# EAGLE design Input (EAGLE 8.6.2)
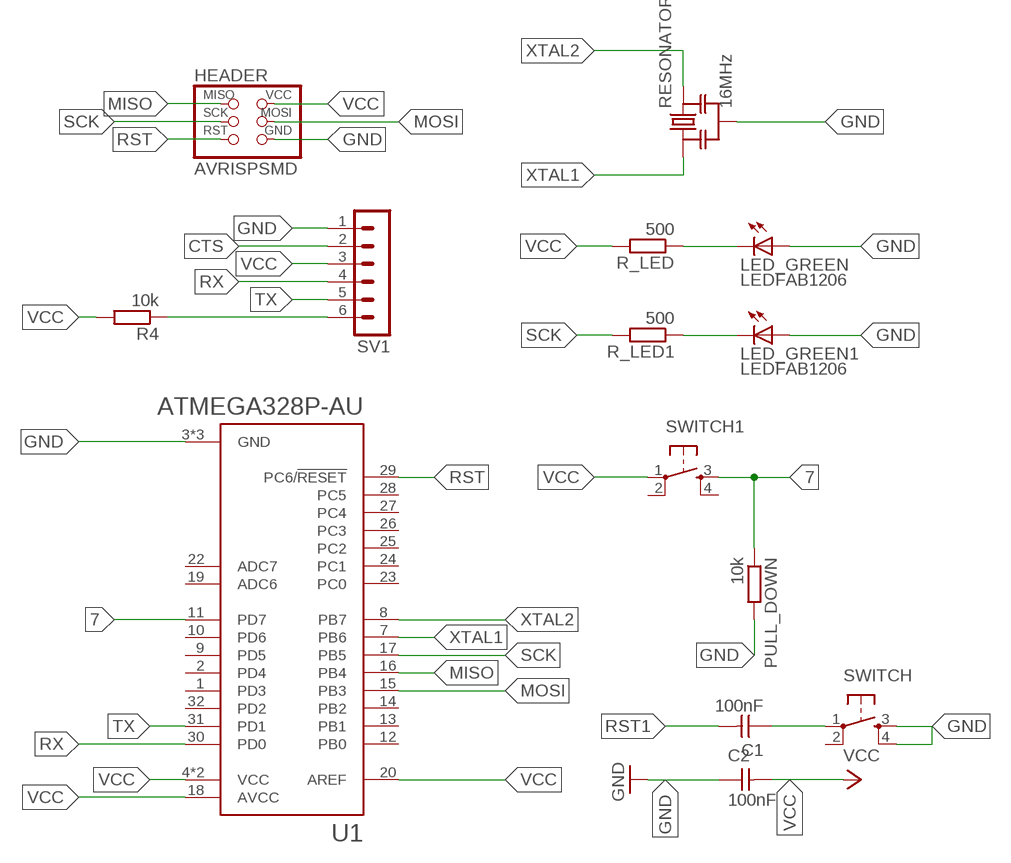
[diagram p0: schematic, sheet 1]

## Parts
C1  100nF  CAP-UNPOLARIZEDFAB  [C1206FAB]
C2  100nF  CAP-UNPOLARIZEDFAB  [C1206FAB]
HEADER  AVRISPSMD  [2X03SMD]
LED_GREEN  LEDFAB1206  [LED1206FAB]
LED_GREEN1  LEDFAB1206  [LED1206FAB]
PULL_DOWN  10k  R-EU_R1206  [R1206]
R4  10k  R-EU_R1206  [R1206]
R_LED  500  R-EU_R1206  [R1206]
R_LED1  500  R-EU_R1206  [R1206]
RESONATOR  16MHz  RESONATOR-MURATACSTCR_G  [RESONATOR_MURATA3]
SV1  MA06-1  [MA06-1]
SWITCH  6MM_SWITCH6MM_SWITCH  [6MM_SWITCH]
SWITCH1  6MM_SWITCH6MM_SWITCH  [6MM_SWITCH]
U1  ATMEGA328P-AU  [QFP80P900X900X120-32N]

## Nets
7: PULL_DOWN.1 SWITCH1.3(S) U1.11(PD7)
CTS: SV1.2
GND: C2.1 HEADER.6(GND) LED_GREEN1.1(A) LED_GREEN.1(A) PULL_DOWN.2 RESONATOR.2 SV1.1 SWITCH.3(S) SWITCH.4(S1) U1.3(GND) U1.5(GND) U1.21(GND)
MISO: HEADER.1(MISO) U1.16(PB4)
MOSI: HEADER.4(MOSI) U1.15(PB3)
N$1: LED_GREEN1.2(C) R_LED1.1
N$21: LED_GREEN.2(C) R_LED.1
RST: C1.1 HEADER.5(RST) SWITCH.1(P) U1.29(PC6/!RESET)
RST1: C1.2 R4.1 SV1.6
RX: SV1.4 U1.30(PD0)
SCK: HEADER.3(SCK) R_LED1.2 U1.17(PB5)
TX: SV1.5 U1.31(PD1)
VCC: C2.2 HEADER.2(VCC) R4.2 R_LED.2 SV1.3 SWITCH1.1(P) U1.4(VCC) U1.6(VCC) U1.18(AVCC) U1.20(AREF)
XTAL1: RESONATOR.1 U1.7(PB6)
XTAL2: RESONATOR.3 U1.8(PB7)
Unconnected: SWITCH1.2(P1) SWITCH1.4(S1) SWITCH.2(P1) U1.1(PD3) U1.2(PD4) U1.9(PD5) U1.10(PD6) U1.12(PB0) U1.13(PB1) U1.14(PB2) U1.19(ADC6) U1.22(ADC7) U1.23(PC0) U1.24(PC1) U1.25(PC2) U1.26(PC3) U1.27(PC4) U1.28(PC5) U1.32(PD2)

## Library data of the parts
C1 C2 = fab:CAP-UNPOLARIZED
HEADER = fab:AVRISP
LED_GREEN LED_GREEN1 = fab:LED: LED
PULL_DOWN R4 R_LED R_LED1 = resistor:R-EU_: RESISTOR, European symbol
RESONATOR = m-pad-2.1:RESONATOR-MURATA: Murata ceramic Resonator "ceralock" CSTCE series with built in load capacitance +- 0.5% tolerance 12.51MHz to 19.99MHz 16MHz murata part#: CSTCE16M0V53-R0 16MHz digikey part#: 490-1198-1-ND $1.33 each
SV1 = con-lstb:MA06-1: PIN HEADER; OC_FARNELL: unknown; OC_NEWARK: unknown
SWITCH SWITCH1 = fab:6MM_SWITCH: OMRON SWITCH
U1 = ATMEGA328P-AU:ATMEGA328P-AU: ATmega Series 20 MHz 32 KB Flash 2 KB SRAM 8-Bit Microcontroller - TQFP-32; AVAILABILITY: Good; DESCRIPTION: ATmega Series 20 MHz 32 KB Flash 2 KB SRAM 8-Bit Microcontroller - TQFP-32; MF: Atmel; MP: ATMEGA328P-AU; PACKAGE: TQFP-32 Atmel; PRICE: 2.38 USD

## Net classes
0 default: clearance 0.205 mm

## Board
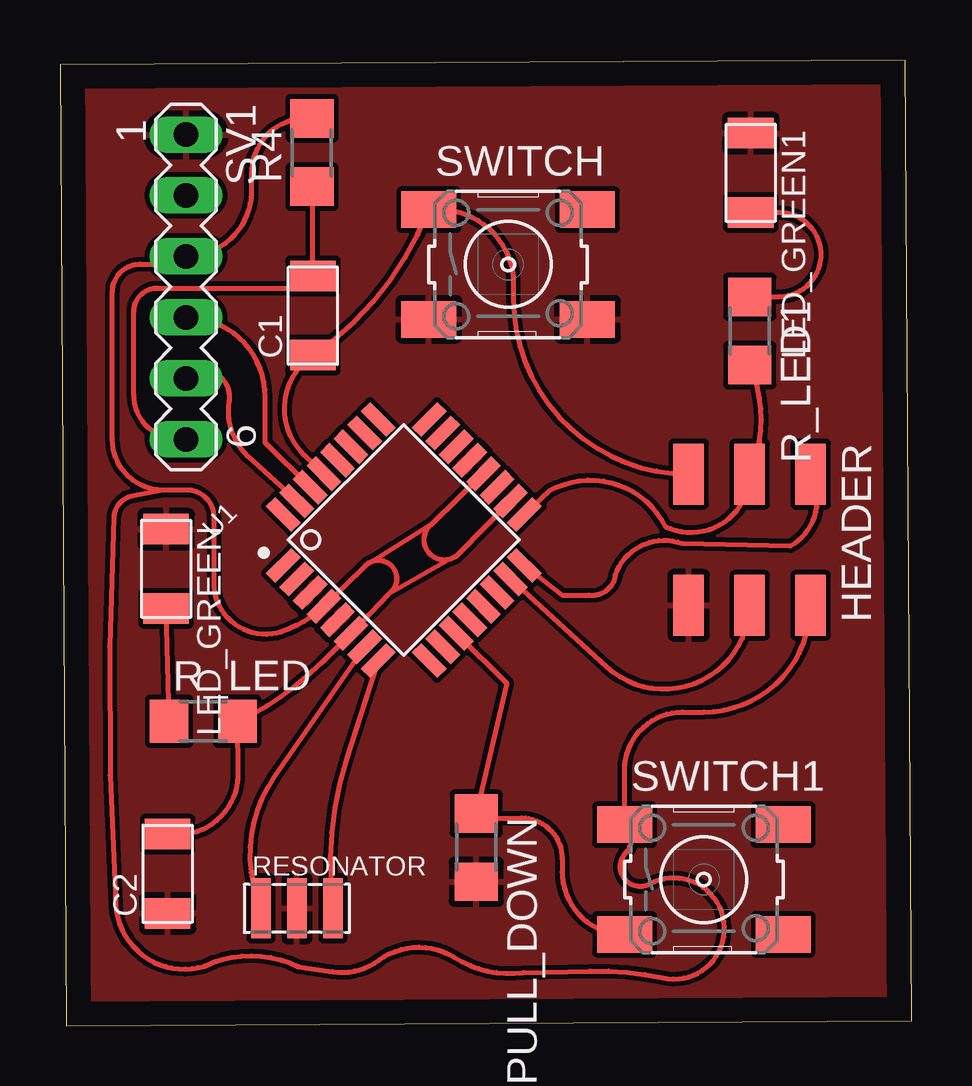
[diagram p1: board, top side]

Size 35.49 x 40.23 mm. Coordinates in mm from the lower left corner, seen from the top.
Outline: 0.27,0 35.49,0.2 35.23,40.23 0,40.03 0.27,0
Copper layers (1*16): Top 0.035mm / dielectric 1.5mm / Bottom 0.035mm
Design rules "default *": minimum track width 6mil, minimum drill 0.35mm, track to track 8mil, track to pad 8mil, pad to pad 8mil, via to via 8mil, smd to smd 8mil, copper to edge 40mil, drill to drill 8mil, minimum pad ring 10mil, minimum via ring 8mil, stop-mask expansion 4mil, vias tented up to drill 0mil, thermal gap 10mil

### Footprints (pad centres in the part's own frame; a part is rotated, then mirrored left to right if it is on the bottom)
C1206FAB = smd 1.27 x 1.905: 1 -1.651,0; 2 1.651,0
2X03SMD = smd 2.54 x 1.27: 1 -2.54,2.54; 2 2.92,2.54; 3 -2.54,0; 4 2.92,0; 5 -2.54,-2.54; 6 2.92,-2.54
LED1206FAB = smd 1.27 x 1.905: 1 -1.651,0; 2 1.651,0
R1206 = smd 1.6 x 1.803: 1 -1.422,0; 2 1.422,0
RESONATOR_MURATA3 = smd 0.8 x 2.5: 1 -1.5,0; 2 0,0; 3 1.5,0
MA06-1 = drill 1.016 long: 1 -6.35,0; 2 -3.81,0; 3 -1.27,0; 4 1.27,0; 5 3.81,0; 6 6.35,0
6MM_SWITCH = smd 2.286 x 1.524: 1 -3.302,2.286; 2 3.302,2.286; 3 -3.302,-2.286; 4 3.302,-2.286
QFP80P900X900X120-32N = smd 1.5 x 0.55: 1 -4.3,2.8; 2 -4.3,2; 3 -4.3,1.2; 4 -4.3,0.4; 5 -4.3,-0.4; 6 -4.3,-1.2; 7 -4.3,-2; 8 -4.3,-2.8; 17 4.3,-2.8; 18 4.3,-2; 19 4.3,-1.2; 20 4.3,-0.4; 21 4.3,0.4; 22 4.3,1.2; 23 4.3,2; 24 4.3,2.8 | smd 0.55 x 1.5: 9 -2.8,-4.3; 10 -2,-4.3; 11 -1.2,-4.3; 12 -0.4,-4.3; 13 0.4,-4.3; 14 1.2,-4.3; 15 2,-4.3; 16 2.8,-4.3; 25 2.8,4.3; 26 2,4.3; 27 1.2,4.3; 28 0.4,4.3; 29 -0.4,4.3; 30 -1.2,4.3; 31 -2,4.3; 32 -2.8,4.3

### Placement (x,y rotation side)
C1  10.54,29.58 90 top
C2  4.48,6.32 90 top
HEADER  28.73,20.43 270 top
LED_GREEN  4.42,19.03 270 top
LED_GREEN1  28.78,35.53 270 top
PULL_DOWN  17.34,7.41 270 top
R4  10.5,36.38 90 top
R_LED  5.97,12.68 0 top
R_LED1  28.74,28.94 270 top
RESONATOR  9.87,4.88 0 top
SV1  5.25,30.78 270 top
SWITCH  18.67,31.71 0 top
SWITCH1  26.83,6.08 0 top
U1  14.32,20.23 45 top

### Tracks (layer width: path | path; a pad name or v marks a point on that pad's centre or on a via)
7
  Top 0.2: U1.11 18.62,14.26 PULL_DOWN.1 17.34,8.65 19.23,8.65 arc-90 20.92,6.96 20.92,6.4 arc90 SWITCH1.3
GND
  pour Top: -54.03,71.48 -54.03,-64.41 -52.76,-65.68 62.81,-65.68 69.16,-59.33 69.16,72.75 59,82.91 -42.6,82.91
MISO
  Top 0.2: U1.16 20.92,17.94 22.04,17.94 arc90 23.15,18.77 23.13,18.77 arc-90 25.94,20.09 30.44,19.99 arc90 HEADER.1
MOSI
  Top 0.2: U1.15 22.77,14.95 arc131 HEADER.4
N$1
  Top 0.2: R_LED1.1 29.97,30.37 arc197 29.44,33.79 arc-50 LED_GREEN1.2
N$21
  Top 0.2: R_LED.1 LED_GREEN.2
RST
  Top 0.2: U1.29 10.2,23.75 arc-102 C1.1 arc34 SWITCH.1 15.8,34 arc-90 18.89,30.91 18.89,30.27 arc90 HEADER.5
RST1
  Top 0.2: R4.1 arc-90 10.54,34.92 C1.2 arc-90 10.03,30.73 4.05,30.73 arc90 3.08,29.75 3.08,26.27 arc90 4.93,24.43 SV1.6
RX
  Top 0.2: U1.30 8.55,24.28 8.55,26.21 arc90 SV1.4
SCK
  Top 0.2: U1.17 20.39,22.27 arc-93 25.22,20.79 arc115 HEADER.3 arc48 R_LED1.2
TX
  Top 0.2: U1.31 7.85,23.71 arc-57 7.06,26.01 arc143 SV1.5
VCC
  Top 0.2: 12.72,19.17 U1.4 arc-27 9.23,16.41 arc-103 6.42,18.28 6.42,21.18 arc90 5.29,22.31 4.29,22.31 | 12.72,19.17 arc-187 13.72,18 | 13.72,18 U1.6 arc-4 10.26,14.54 arc-18 R_LED.2 7.42,10.5 arc-100 C2.2 | U1.20 15.53,20.93 | U1.18 16.62,19.65 | 16.62,19.65 arc-190 15.53,20.93 | 12.72,19.17 15.53,20.93 | 13.72,18 16.62,19.65 | R4.2 10.27,37.8 arc90 7.97,35.5 7.97,34.77 arc-90 SV1.3 arc-90 4.93,31.72 3.34,31.72 arc90 2.18,30.57 2.18,24.42 arc90 4.29,22.31 | HEADER.2 arc-90 26.82,13.06 25.94,13.06 arc90 23.53,10.65 SWITCH1.1 arc-94 23.58,7.2 arc163 24.58,5.89 arc-221 25.13,1.98 arc14 22.09,2.27 19.31,2.2 arc-39 16.43,2.84 arc68 13.28,2.72 arc-45 11.35,2.24 9.93,2.45 arc51 6.02,2.48 arc-104 2.32,5.03 arc-6 2.24,21.18 arc-76 3,22.06 4.29,22.31
XTAL1
  Top 0.2: U1.7 8.93,10.36 arc58 RESONATOR.1
XTAL2
  Top 0.2: U1.8 11.95,11.13 arc25 RESONATOR.3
